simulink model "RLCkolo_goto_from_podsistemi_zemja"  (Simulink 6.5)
settings: Solver=ode45  StartTime=0.0  StopTime=1  RelTol=1e-6
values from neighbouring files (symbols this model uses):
  A = [-R/L -1/L; 1/C 0]    [primer_7_4c.m]
  C = str2num(C)    [patuvacki_bran_1.m]    (also in primer_7_3.m = 0.0001; primer_7_4.m = 0.0001; primer_7_4a.m = 0.0001; primer_7_4c.m = 0.0001)
undefined symbols (not defined in the file or in its folder): B, blocks, Continuous, D, powergui, x0, ZData
libraries: powerlib x8

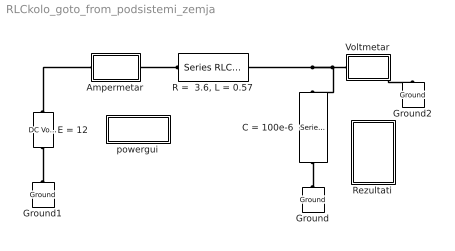
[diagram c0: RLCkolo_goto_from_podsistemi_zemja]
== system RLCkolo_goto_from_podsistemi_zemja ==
  Ampermetar : Subsystem
  C = 100e-6 : powerlib/Elements/Series RLC Branch  Orientation=down  DialogController=PMDialogs.PMDefaultMaskDlg  PhysicalDomain=powersysdomain  SubClassName=unknown  LeftPortType=p1  RightPortType=p1  LConnTagsString=__new0  RConnTagsString=__new0  BranchType=C  Resistance=1  Inductance=1e-3  SetiL0=off  InitialCurrent=0  Capacitance=100e-6  Setx0=on  InitialVoltage=0  Measurements=Branch voltage
  E = 12 : powerlib/Electrical Sources/DC Voltage Source  Orientation=up  DialogController=PMDialogs.PMDefaultMaskDlg  SystemSampleTime=-1  Amplitude=12  Measurements=None
  Ground : powerlib/Elements/Ground  Orientation=down  DialogController=PMDialogs.PMDefaultMaskDlg  PhysicalDomain=powersysdomain  SubClassName=unknown  LeftPortType=p1  RightPortType=p1  LConnTagsString=a
  Ground1 : powerlib/Elements/Ground  Orientation=down  DialogController=PMDialogs.PMDefaultMaskDlg  PhysicalDomain=powersysdomain  SubClassName=unknown  LeftPortType=p1  RightPortType=p1  LConnTagsString=a
  Ground2 : powerlib/Elements/Ground  Orientation=down  DialogController=PMDialogs.PMDefaultMaskDlg  PhysicalDomain=powersysdomain  SubClassName=unknown  LeftPortType=p1  RightPortType=p1  LConnTagsString=a
  "R =  3.6, L = 0.57" : powerlib/Elements/Series RLC Branch  DialogController=PMDialogs.PMDefaultMaskDlg  PhysicalDomain=powersysdomain  SubClassName=unknown  LeftPortType=p1  RightPortType=p1  LConnTagsString=__new0  RConnTagsString=__new0  BranchType=RL  Resistance=3.6  Inductance=0.57  SetiL0=on  InitialCurrent=0  Capacitance=100e-6  Setx0=on  InitialVoltage=0  Measurements=Branch current
  Rezultati : Subsystem
  Voltmetar : Subsystem
  powergui : Subsystem  AncestorBlock=powerlib/powergui  InitFcn=powergui( 'InitFcn_Callback' , gcb , 0 , [ ] );  mask(PSB option menu block){SimulationMode=Continuous, SampleTime=50e-6, echomessages=off, RestoreLinks=warning, x0status=blocks, Frange=[0:2:500], Ylog=off, Xlog=on, ShowGrid=off, save=off, variable=ZData, structure=, ZoomFFT=on, StartTime=0.0, cycles=1, DisplayStyle=1, fundamental=60, FreqAxis=off, MaxFrequency=1000, frequencyindice=0, frequencyindicesteady=1, RmsSteady=1, display=off, Ts=0, frequency=60, methode=off, HookPort=off, Interpol=off}
      mask prompts: SimulationMode "Simulation mode"; SampleTime "Sample time Ts (when simulation mode is Discrete) (s)"; echomessages "Echo  Messages"; RestoreLinks "Restore disabled links"; x0status "Initial electrical states status"; Frange "Impedance tool: Frequency Range"; Ylog "Impedance tool: Log impedance"; Xlog "Impedance tool: log Frequency"; ShowGrid "Impedance tool: grid"; save "Impedance tool: Save Data To Workspace"; variable "Impedance tool: Variable Name"; structure "Structure Name (PSBFFTSCOPE)"; ZoomFFT "ZoomFFT (PSBFFTSCOPE)"; StartTime "Start Time (PSBFFTSCOPE)"; cycles "Cycles (PSBFFTSCOPE)"; DisplayStyle "Display style (PSBFFTSCOPE)"; fundamental "Fundamental (PSBFFTSCOPE)"; FreqAxis "Frequency Axis (PSBFFTSCOPE)"; MaxFrequency "Max Frequency (PSBFFTSCOPE)"; frequencyindice "Load flow frequency (Hz)"; frequencyindicesteady "Frequency indice (STEADYSTATE)"; RmsSteady "RMS display (STEADYSTATE)"; display "Display Results"; Ts "OBSOLETE 1"; frequency "Phasor frequency (Hz)"; methode "Phasor simulation"; HookPort "Hook port"; Interpol "Interpolate"
      mask init:
      | powerlibroot = which('powersysdomain');
      | PSBroot = powerlibroot(1:end-16);
      | %
      | switch SimulationMode
      | 	case 1
      | 		message=sprintf('Continuous');
      | 	case 2
      |         SampleTimeeval=evalin('base',SampleTime,'NaN');
      |         if isnan(SampleTimeeval)
      |             message=sprintf('Warning !!,\nUndefined sample time');
      |         else
      |             message=sprintf('Discrete,\nTs = %.4g s.',SampleTimeeval);
      |         end
      | 	case 3
      | 		message=sprintf('Phasors');
      | end
      | if strcmp(bdroot,'powerlib')
      |   message='powergui';
      | end
      | power_initmask();
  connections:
  Voltmetar/LConn1 -- "R =  3.6, L = 0.57"/RConn1 -- C = 100e-6/LConn1
  E = 12/RConn1 -- Ampermetar/LConn1
  Ampermetar/RConn1 -- "R =  3.6, L = 0.57"/LConn1
  Ground/LConn1 -- C = 100e-6/RConn1
  Ground1/LConn1 -- E = 12/LConn1
  Voltmetar/RConn1 -- Ground2/LConn1

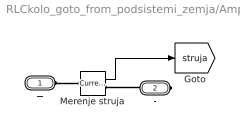
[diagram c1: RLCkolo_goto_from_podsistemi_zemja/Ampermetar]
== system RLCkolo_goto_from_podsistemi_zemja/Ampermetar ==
  Merenje struja : powerlib/Measurements/Current Measurement  DialogController=PMDialogs.PMDefaultMaskDlg  SystemSampleTime=-1  PhasorSimulation=off  OutputType=Complex  PSBequivalent=0
  + : PMIOPort  Port=1  Side=Left
  - : PMIOPort  Orientation=left  Port=2  Side=Right
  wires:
  Merenje struja/1 -> [struja]
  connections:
  +/RConn1 -- Merenje struja/LConn1
  -/RConn1 -- Merenje struja/RConn1

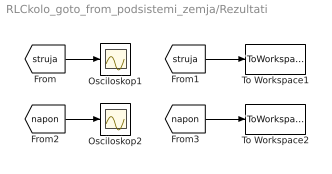
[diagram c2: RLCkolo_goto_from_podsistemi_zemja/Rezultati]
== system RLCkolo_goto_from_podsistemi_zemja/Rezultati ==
  Osciloskop1 : Scope
  Osciloskop2 : Scope
  To Workspace1 : ToWorkspace  VariableName=napon  SampleTime=-1  SaveFormat=Array
  To Workspace2 : ToWorkspace  VariableName=struja  SampleTime=-1  SaveFormat=Array
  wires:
  [struja] -> Osciloskop1/1
  [struja] -> To Workspace1/1
  [napon] -> Osciloskop2/1
  [napon] -> To Workspace2/1

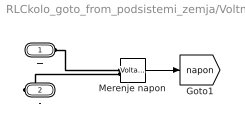
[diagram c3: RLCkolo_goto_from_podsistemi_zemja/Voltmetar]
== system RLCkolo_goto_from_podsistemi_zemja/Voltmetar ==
  Merenje napon : powerlib/Measurements/Voltage Measurement  DialogController=PMDialogs.PMDefaultMaskDlg  SystemSampleTime=-1  PhasorSimulation=off  OutputType=Complex  PSBequivalent=0
  + : PMIOPort  Port=1  Side=Left
  - : PMIOPort  Port=2  Side=Right
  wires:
  Merenje napon/1 -> [napon]
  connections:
  +/RConn1 -- Merenje napon/LConn1
  -/RConn1 -- Merenje napon/LConn2

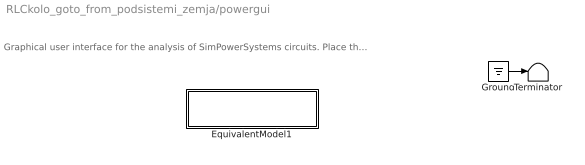
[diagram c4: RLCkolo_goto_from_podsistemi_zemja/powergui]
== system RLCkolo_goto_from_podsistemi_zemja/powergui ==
  note: Graphical user interface for the analysis of SimPowerSystems circuits. Place the Powergui block in the top-level of your model and double-click on it to open the GUI.
  EquivalentModel1 : Subsystem
  Ground : Ground
  Terminator : Terminator
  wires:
  Ground/1 -> Terminator/1

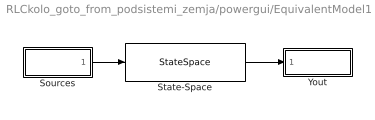
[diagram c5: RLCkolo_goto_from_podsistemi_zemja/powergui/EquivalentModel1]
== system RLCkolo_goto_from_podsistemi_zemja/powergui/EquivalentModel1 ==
  Sources : Subsystem
  State-Space : StateSpace  A=A  B=B  C=C  D=D  X0=x0
  Yout : Subsystem
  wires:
  Sources/1(u) -> State-Space/1
  State-Space/1 -> Yout/1(v,i)

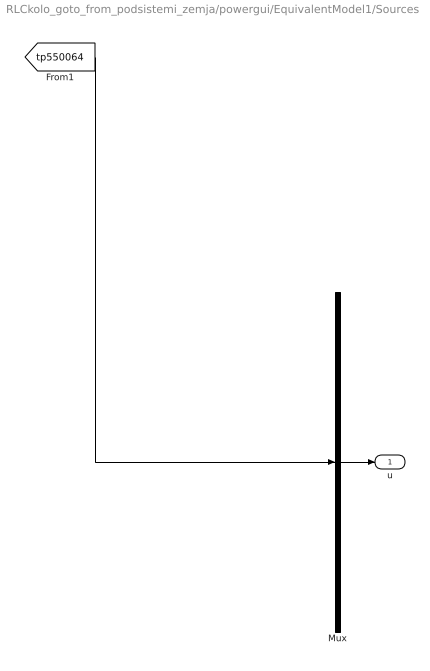
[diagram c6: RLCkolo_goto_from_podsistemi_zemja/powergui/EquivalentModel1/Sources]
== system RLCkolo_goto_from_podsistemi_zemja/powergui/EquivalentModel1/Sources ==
  Mux : Mux  Inputs=1
  u : Outport
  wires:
  Mux/1 -> u/1
  [tp550064] -> Mux/1

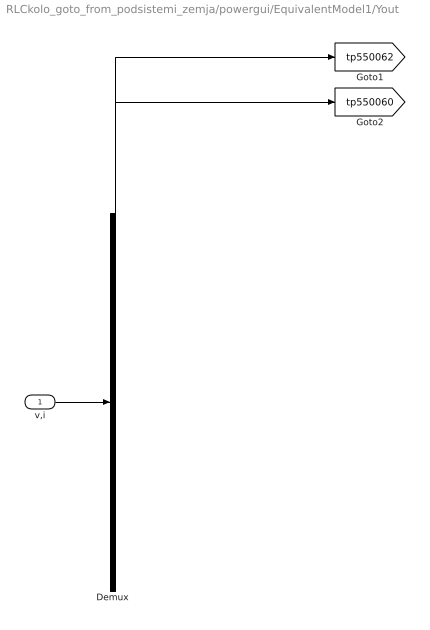
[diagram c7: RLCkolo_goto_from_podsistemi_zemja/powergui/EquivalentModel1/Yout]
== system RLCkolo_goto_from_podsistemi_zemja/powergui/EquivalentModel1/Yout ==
  v,i : Inport
  Demux : Demux  Outputs=[1 1]
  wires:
  v,i/1 -> Demux/1
  Demux/1 -> [tp550062]
  Demux/2 -> [tp550060]
